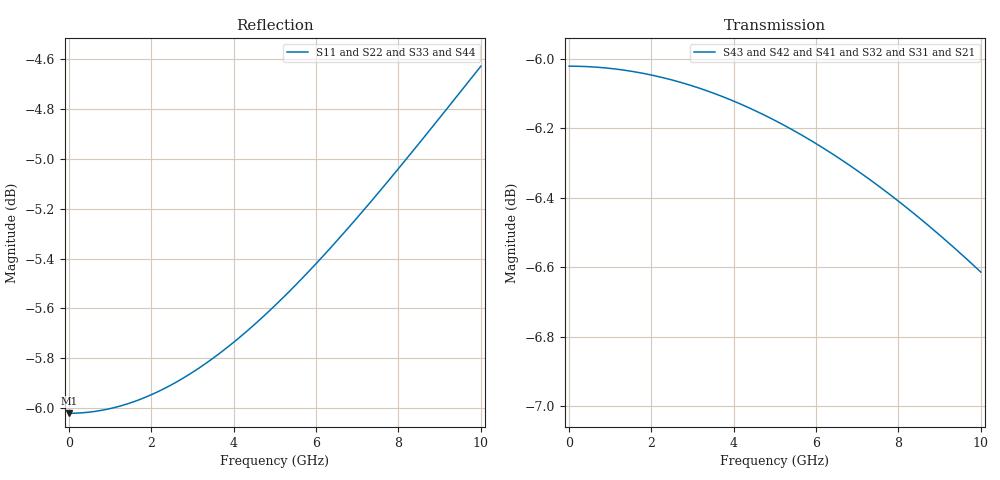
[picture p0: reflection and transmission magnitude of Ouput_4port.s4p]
! Created Tue Nov 10 09:05:16 2020
# ghz S ma R 50
! 4 Port Network Data from SP1.SP block
! freq  magS11  angS11  magS12  angS12  magS13  angS13  magS14  angS14
!  magS21  angS21  magS22  angS22  magS23  angS23  magS24  angS24
!  magS31  angS31  magS32  angS32  magS33  angS33  magS34  angS34
!  magS41  angS41  magS42  angS42  magS43  angS43  magS44  angS44
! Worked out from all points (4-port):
!   1000 points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, 10 MHz to 10 GHz, reference 50 ohm
!   strongest paths, dB at 10 MHz, 2.51 GHz, 5.01 GHz, 7.51 GHz, 10 GHz:
!     S43: -6.0, -6.1, -6.2, -6.4, -6.6
!     S42: -6.0, -6.1, -6.2, -6.4, -6.6
!     S41: -6.0, -6.1, -6.2, -6.4, -6.6
!     S32: -6.0, -6.1, -6.2, -6.4, -6.6
!     S31: -6.0, -6.1, -6.2, -6.4, -6.6
!     S21: -6.0, -6.1, -6.2, -6.4, -6.6
!   lowest |S11| = -6.0 dB at 10 MHz (marker M1), VSWR 3.00, Z = 16.7 - j0.00842 ohm
!   |S11| at or under -10 dB: nowhere
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0.01  0.5 -180.0  0.5 -0.0  0.5 -0.0  0.5 -0.0
      0.5 -0.0  0.5 -180.0  0.5 -0.0  0.5 -0.0
      0.5 -0.0  0.5 -0.0  0.5 -180.0  0.5 -0.0
      0.5 -0.0  0.5 -0.0  0.5 -0.0  0.5 -180.0
1.11  0.5013 -177.6  0.4995 -2.4  0.4995 -2.4  0.4995 -2.4
      0.4995 -2.4  0.5013 -177.6  0.4995 -2.4  0.4995 -2.4
      0.4995 -2.4  0.4995 -2.4  0.5013 -177.6  0.4995 -2.4
      0.4995 -2.4  0.4995 -2.4  0.4995 -2.4  0.5013 -177.6
2.23  0.5053 -175.2  0.4982 -4.8  0.4982 -4.8  0.4982 -4.8
      0.4982 -4.8  0.5053 -175.2  0.4982 -4.8  0.4982 -4.8
      0.4982 -4.8  0.4982 -4.8  0.5053 -175.2  0.4982 -4.8
      0.4982 -4.8  0.4982 -4.8  0.4982 -4.8  0.5053 -175.2
3.39  0.5121 -172.9  0.4958 -7.3  0.4958 -7.3  0.4958 -7.3
      0.4958 -7.3  0.5121 -172.9  0.4958 -7.3  0.4958 -7.3
      0.4958 -7.3  0.4958 -7.3  0.5121 -172.9  0.4958 -7.3
      0.4958 -7.3  0.4958 -7.3  0.4958 -7.3  0.5121 -172.9
4.63  0.522 -170.6  0.4923 -9.9  0.4923 -9.9  0.4923 -9.9
      0.4923 -9.9  0.522 -170.6  0.4923 -9.9  0.4923 -9.9
      0.4923 -9.9  0.4923 -9.9  0.522 -170.6  0.4923 -9.9
      0.4923 -9.9  0.4923 -9.9  0.4923 -9.9  0.522 -170.6
7.43  0.5526 -166.4  0.4809 -15.7  0.4809 -15.7  0.4809 -15.7
      0.4809 -15.7  0.5526 -166.4  0.4809 -15.7  0.4809 -15.7
      0.4809 -15.7  0.4809 -15.7  0.5526 -166.4  0.4809 -15.7
      0.4809 -15.7  0.4809 -15.7  0.4809 -15.7  0.5526 -166.4
10  0.5869 -163.7  0.467 -20.7  0.467 -20.7  0.467 -20.7
    0.467 -20.7  0.5869 -163.7  0.467 -20.7  0.467 -20.7
    0.467 -20.7  0.467 -20.7  0.5869 -163.7  0.467 -20.7
    0.467 -20.7  0.467 -20.7  0.467 -20.7  0.5869 -163.7
